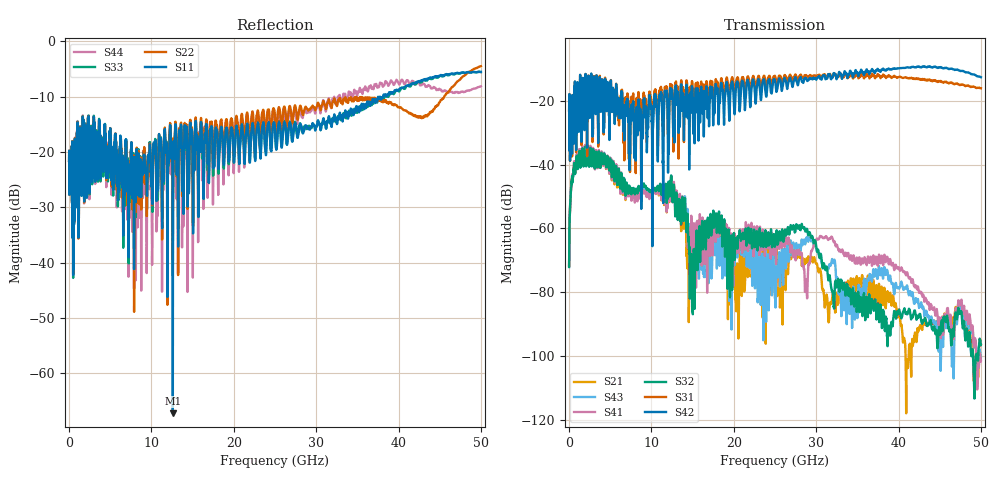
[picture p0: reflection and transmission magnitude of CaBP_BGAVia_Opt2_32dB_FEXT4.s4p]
!* Samtec Inc. NovaRay Examax Flyover System  *
!*  REV DATE  = 08/08/18  *
!*  TYPE  = TOUCHSTONE  *
!*  PORTS  = 4 port  *
!*  UNITS  = GHz  *
!*  DATA RANGE = DC  to 50 GHz; 10 MHz Step  *
!*  PARAMETER  = S  *
!*  FORMAT  = Real-Imaginary  *
!*  REFERENCE  = 50 ohms  *
!*  SOURCE  = HFSS  *
!*  VALIDATED  = No  *
!*  MANUFACTURER = SAMTEC  *
!*  INTERCONNECT = NVAx to EBCx to EBCx to NVAx  *
!*  [Full Channel NVAx to EBCx to EBCx to NVAx  with PCB Trace and BGA Via]  *
!*  BOUNDARY A  = Silicon BGA Ball Pad  *
!*  BOUNDARY B  = Silicon BGA Ball Pad  *
!*  NVAx (end a) ->>- (end b) NVAx  *
!*  Port 01 ->>- Port 02  *
!*  Port 03 ->>- Port 04  *
!***************************** CHANNEL MODEL ******************************************
# GHz S RI R 50
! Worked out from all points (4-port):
!   5000 points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, 10 MHz to 50 GHz, reference 50 ohm
!   strongest paths, dB at 10 MHz, 12.51 GHz, 25.01 GHz, 37.51 GHz, 50 GHz:
!     S42: -23.1, -16.6, -13.7, -10.1, -12.6
!     S31: -23.1, -15.2, -12.2, -11.7, -16.1
!     S32: -72.1, -48.4, -65.2, -83.7, -96.5
!     S41: -71.5, -47.8, -65.9, -71.2, -101.6
!     S43: -71.7, -47.8, -81.9, -74.7, -100.4
!     S21: -71.7, -48.5, -67.9, -81.6, -96.6
!   lowest |S11| = -67.2 dB at 12.6 GHz (marker M1), VSWR 1.00, Z = 50 + j0.0147 ohm
!   |S11| at or under -10 dB: start of sweep to 37.74 GHz; 37.74 GHz to 38.13 GHz (385.5 MHz wide, 1.02 % of centre); 38.51568 GHz to 38.54961 GHz (33.93 MHz wide, 0.0881 % of centre)
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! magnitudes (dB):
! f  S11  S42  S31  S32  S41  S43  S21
! 10 MHz  -21.6  -23.1  -23.1  -72.1  -71.5  -71.7  -71.7
! 1.41 GHz  -17.5  -14.3  -14.4  -39.0  -38.5  -38.7  -38.7
! 12.6 GHz  -67.2  -22.3  -21.8  -49.6  -49.0  -49.0  -49.8
! 14.88 GHz  -16.0  -16.5  -15.1  -77.7  -59.4  -60.5  -69.6
! 17.66 GHz  -20.7  -23.3  -18.9  -59.2  -58.3  -66.9  -60.7
! 20.42 GHz  -16.0  -14.1  -12.8  -65.9  -63.0  -69.1  -72.2
! 50 GHz  -5.5  -12.6  -16.1  -96.5  -101.6  -100.4  -96.6
